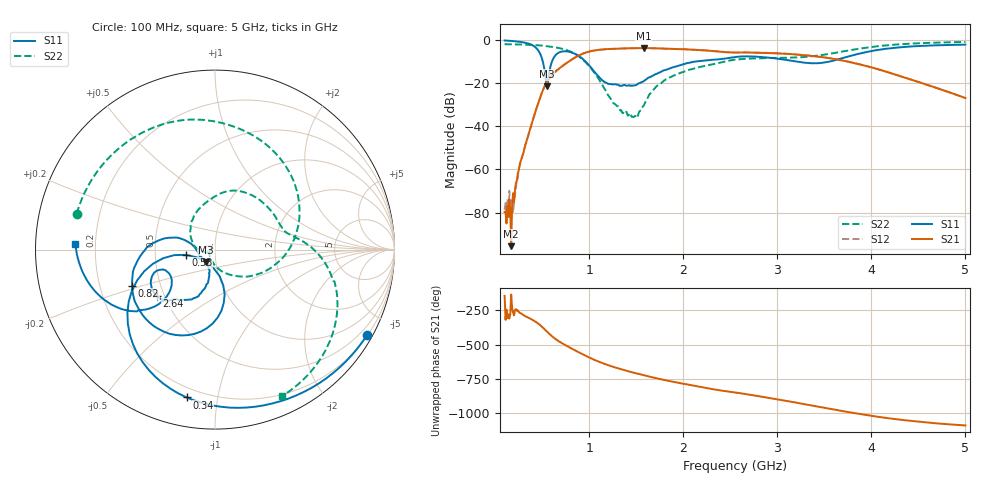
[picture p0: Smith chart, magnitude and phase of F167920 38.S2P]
!  2-Port S-parameters saved by WinCal
! VAR MeasName=S-Parameters (CALIBRATED_DATA) read from VNA (N5242A)
! VAR MeasDate=2016-11-22 9:57:17
! VAR NAME=F167920 38
! VAR FILENAME=F167920 38.S2P
! VAR DATE=2016-11-22 9:57:17
! VAR PHYS_PORTS=1,2
# Hz S DB R 50
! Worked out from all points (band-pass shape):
!   491 points, 100 MHz to 5 GHz, reference 50 ohm
!   highest |S21| = -3.77 dB at 1.58 GHz (marker M1); lowest = -95.5 dB at 170 MHz (marker M2)
!   |S21| within 3 dB of the highest: 910.3 MHz to 3.207 GHz (2.297 GHz wide, 112 % of centre)
!   lowest |S11| = -21.4 dB at 550 MHz (marker M3), VSWR 1.19, Z = 44.8 - j6.16 ohm
!   |S11| at or under -10 dB: 505.8 MHz to 603.9 MHz (98.09 MHz wide, 17.7 % of centre); 959.1 MHz to 2.134 GHz (1.175 GHz wide, 76 % of centre); 3.2 GHz to 3.558 GHz (357.2 MHz wide, 10.6 % of centre)
!   |S22| runs from -36.1 to -0.9 dB; largest |S21 - S12| = 0.002
!   S11 on the Smith chart (normalised r, x): 100 MHz: 0.22, -3.82; 340 MHz: 0.15, -0.82; 530 MHz: 0.72, -0.04; 820 MHz: 0.34, -0.19; 2.64 GHz: 0.45, -0.28; 5 GHz: 0.12, +0.02
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1e8  -0.25 -29.3  -79.72 -143.8  -78.67 126.7  -1.98 165.5
1.7e8  -0.47 -49.3  -95.54 -133.9  -82.25 37.0  -2.03 155.2
1.9e8  -0.54 -55.1  -71.02 95.3  -80.03 122.2  -2.04 152.3
2.7e8  -0.94 -78.6  -56.20 90.1  -56.30 88.6  -2.12 140.1
3.4e8  -1.53 -100.8  -45.89 62.0  -46.01 64.5  -2.22 129.0
4.5e8  -4.42 -144.2  -30.26 18.5  -30.27 18.3  -2.46 110.1
5.3e8  -15.61 -169.9  -21.06 -30.0  -21.07 -29.9  -2.79 94.9
5.5e8  -21.43 -126.4  -19.43 -43.5  -19.43 -43.5  -2.90 90.9
6.5e8  -6.68 -99.8  -14.32 -101.9  -14.32 -101.9  -3.54 69.7
8.2e8  -5.95 -156.3  -8.93 -169.8  -8.92 -169.9  -5.77 23.7
9.2e8  -8.40 178.3  -6.56 154.7  -6.54 154.7  -8.66 -9.3
1.11e9  -17.45 166.7  -4.54 94.9  -4.53 94.9  -18.78 -77.1
1.34e9  -21.19 -148.2  -3.95 41.7  -3.95 41.7  -32.56 159.4
1.49e9  -20.97 -122.4  -3.82 13.9  -3.82 13.9  -35.21 164.4
1.58e9  -19.03 -107.2  -3.77 -1.8  -3.77 -1.9  -30.36 -163.7
1.74e9  -15.18 -101.9  -3.94 -27.4  -3.94 -27.4  -20.73 179.2
2.1e9  -10.20 -115.8  -4.51 -76.9  -4.49 -76.9  -13.44 125.0
2.55e9  -7.93 -135.4  -5.83 -126.7  -5.81 -126.8  -9.15 70.2
2.64e9  -7.63 -141.6  -5.80 -136.0  -5.78 -136.1  -8.80 59.2
3.37e9  -10.82 -152.0  -7.43 137.7  -7.40 137.6  -7.56 12.2
4.19e9  -3.93 -150.0  -15.17 44.5  -15.14 44.1  -2.39 -26.3
5e9  -2.17 177.5  -26.94 -7.2  -26.97 -7.6  -0.94 -65.5
